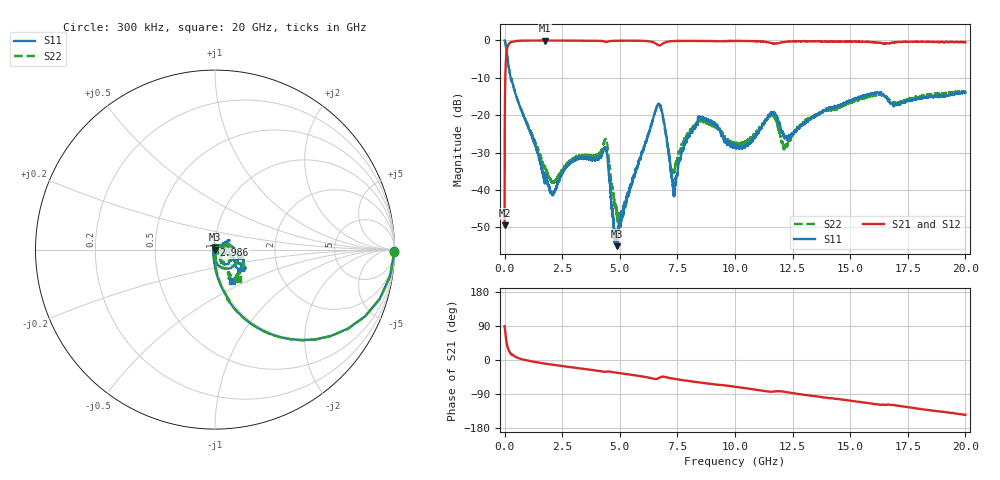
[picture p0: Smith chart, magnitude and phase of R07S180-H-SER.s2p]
!{R07S180}
!Johanson Technology Inc.
!www.johansontechnology.com
!Test Board Conditions:
!Substrate Type  RO4350B
!Substrate Thickness  10 mil
!Substrate Dk  3.66
!TL Type: GCPW
!TL Trace Width  21 mil
!TL Gap  20 mil
!Electrode orientation  Horizontal
!DUT TOPOLOGY	SERIES
!Mounting Pad LxW  16x21 mil
! Created Sat Feb  6 11:49:03 2021
# hz S ma R 50
! 2 Port Network Data from SP1.SP block
! freq  magS11  angS11  magS21  angS21  magS12  angS12  magS22  angS22
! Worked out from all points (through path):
!   20001 points, 300 kHz to 20 GHz, reference 50 ohm
!   highest |S21| = -0.01 dB at 1.755 GHz (marker M1); lowest = -49.5 dB at 300 kHz (marker M2)
!   group delay of S21, straight-line fit = 20.9 ps
!   lowest |S11| = -55.1 dB at 4.871 GHz (marker M3), VSWR 1.00, Z = 50.2 - j0.0694 ohm
!   |S11| at or under -10 dB: 264.6 MHz to end of sweep
!   |S22| runs from -48.5 to 0.0 dB; largest |S21 - S12| = 0.013
!   S11 on the Smith chart (normalised r, x): 300 kHz: open; 2.986 GHz: 0.99, +0.05; 20 GHz: 1.13, -0.42
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300000  0.9993 -0.5  0.003368 89.0  0.003533 88.2  1 -0.7
1.023e8  0.6555 -49.6  0.7505 40.7  0.7522 40.6  0.6573 -49.6
1.763e8  0.4499 -64.7  0.8891 25.7  0.8902 25.8  0.4496 -64.7
1.7553e9  0.01688 -123.0  0.9985 -9.6  0.9976 -9.6  0.02021 -73.3
2.0953e9  0.008454 174.5  0.9975 -12.6  0.9976 -12.6  0.01291 -29.8
2.9863e9  0.02509 103.1  0.996 -19.9  0.9956 -19.8  0.02621 25.8
3.3343e9  0.0268 97.4  0.9948 -22.6  0.9952 -22.6  0.02889 25.6
4.3763e9  0.03645 9.6  0.9574 -31.1  0.9579 -31.0  0.04769 -2.9
4.7103e9  0.004127 -80.7  0.9885 -32.2  0.9878 -32.3  0.009147 -44.7
4.8713e9  0.001763 -23.1  0.9902 -33.7  0.9905 -33.7  0.004702 -18.7
5.0883e9  0.004934 -0.1  0.9918 -35.5  0.9916 -35.5  0.004637 31.0
6.6673e9  0.1406 -26.1  0.8636 -48.7  0.8643 -48.8  0.1371 -26.6
6.8913e9  0.0904 -77.7  0.9199 -44.1  0.9195 -44.0  0.08496 -78.3
7.3403e9  0.008793 -28.2  0.9799 -49.4  0.9805 -49.5  0.01705 -24.0
7.7593e9  0.03529 38.3  0.986 -53.4  0.9862 -53.4  0.04226 17.4
8.4873e9  0.09286 34.2  0.9837 -59.4  0.9838 -59.5  0.08476 26.0
1.00003e10  0.03935 38.1  0.985 -70.7  0.9861 -70.7  0.03904 -18.0
1.16103e10  0.1087 -36.3  0.9164 -83.6  0.917 -83.7  0.1003 -35.8
1.21893e10  0.05196 -51.2  0.959 -84.4  0.9585 -84.4  0.03877 -26.4
1.33343e10  0.09127 -19.7  0.9752 -94.5  0.9762 -94.6  0.09517 2.0
1.66673e10  0.1525 -40.0  0.9098 -117.6  0.9135 -118.0  0.1644 -59.7
2e10  0.202 -61.4  0.9522 -144.8  0.9451 -144.7  0.2078 -53.0
